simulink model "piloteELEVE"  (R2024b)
settings: Solver=ode45  StartTime=0.0  StopTime=35*45*12  RelTol=1e-3  EnableMultiTasking=on
PreLoadFcn:
  | M=0
InitFcn:
  | modelename = gcs
  | path = strcat(gcs,'/mecanisme pilote/Mass')
  | if M==0
  |     set_param(path,'Commented','on')
  | else
  |     set_param(path,'Commented','off')
  | end
libraries: fl_lib x14, nesl_utility x5, sdl_lib x1

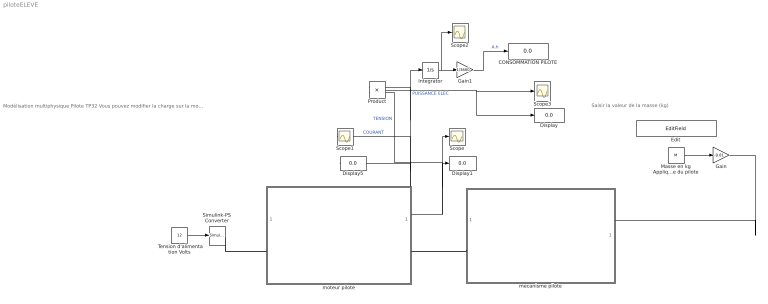
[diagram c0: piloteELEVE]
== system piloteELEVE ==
  note: Saisir la valeur de la masse (kg)
  note: Modélisation multiphysique Pilote TP32 Vous pouvez modifier la charge sur la motorisation du pilote en modifiant la valeur de la masse appliquée sur la tige du pilote.
  " Tension d'alimentation Volts" : Constant  Value=12
  CONSOMMATION PILOTE : Display
  Display : Display
  Display1 : Display
  Display5 : Display
  Edit : EditField  LabelPosition=Hide  ShowInitialText=on  Alignment=Center
  Gain : Gain  Gain=-9.81
  Gain1 : Gain  Gain=1/3600
  Integrator : Integrator
  Masse en kg Appliquée sur la tige en sortie du pilote : Constant  Value=M
  Product : Product
  Scope{,1..3} (4 alike) : Scope
  Simulink-PS Converter : nesl_utility/Simulink-PS Converter  PhysicalDomain=network_engine_domain  SubClassName=ps_input  LeftPortType=input  RightPortType=output  PseudoPeriodic=off  Frequencies=[]  NoiseDistribution=none  NoiseParameters=[]  Unit=1  AffineConversion=off  FilteringAndDerivatives=zero  SimscapeFilterOrder=1  InputFilterTimeConstant=0.001  UdotUserProvided=1
  mecanisme pilote : Subsystem
  moteur pilote : Subsystem
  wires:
  " Tension d'alimentation Volts"/1 -> Simulink-PS Converter/1
  Masse en kg Appliquée sur la tige en sortie du pilote/1 -> Gain/1
  Gain/1 -> mecanisme pilote/1(Masse accrochée sur la tige)
  Integrator/1 -> Scope2/1, Gain1/1
  Product/1 -> Display/1, Scope3/1  "PUISSANCE ELEC"
  Gain1/1 -> CONSOMMATION PILOTE/1  "A.h"
  moteur pilote/2(TENSION) -> Display1/1, Scope/1, Product/2  "TENSION"
  moteur pilote/1(COURANT) -> Display5/1, Integrator/1, Product/1, Scope1/1  "COURANT"
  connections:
  Simulink-PS Converter/RConn1 -- moteur pilote/LConn1
  moteur pilote/RConn1 -- mecanisme pilote/LConn1

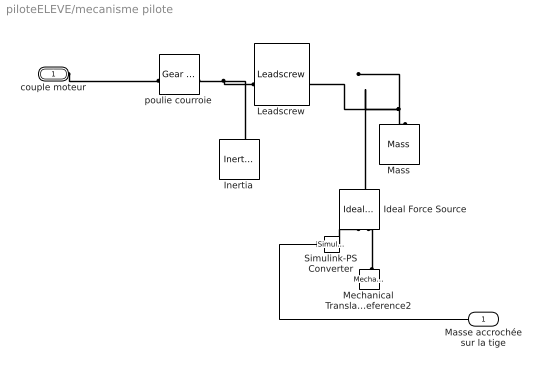
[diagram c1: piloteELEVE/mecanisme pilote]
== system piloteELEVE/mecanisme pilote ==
  Masse accrochée sur la tige : Inport
  Ideal Force Source : fl_lib/Mechanical/Mechanical Sources/Ideal Force Source
  Inertia : fl_lib/Mechanical/Rotational Elements/Inertia  inertia=0.0015 kg*m^2  num_ports=foundation.enum.numPorts2.one  w_specify=off  w_priority=High  w=0 rad/s  w_nominal_specify=off  w_nominal_value=1  w_nominal_unit=rad/s  t_specify=off  t_priority=None  t=0 N*m  t_nominal_specify=off  t_nominal_value=1  t_nominal_unit=N*m
  Leadscrew : sdl_lib/Gears/Rotational- Translational/Leadscrew  Lead=0.003 m  helix_type=sdl.enum.handedness.right  friction_model=sdl.enum.gear_friction.constant  friction_parameterization=sdl.enum.frictionParameterization.geometry  lambda=15 deg  alpha=14.5 deg  fr_coeff=0.25  eff_sn=0.75  eff_ns=0.45  temperature_TLU=[280, 300, 320] K  efficiency_sn_TLU=[.75, .65, .6]  efficiency_ns_TLU=[.5, .45, .4]  pwr_thr=0.001 W  mu_visc=0.0008 N*m*s/rad  thermal_mass=50 J/K  temperature_specify=off  temperature_priority=High  temperature=300 K  temperature_nominal_specify=off  temperature_nominal_value=1  temperature_nominal_unit=K
  Mass : fl_lib/Mechanical/Translational Elements/Mass  mass=M kg  num_ports=foundation.enum.numPorts2.one  v_specify=off  v_priority=High  v=0 m/s  v_nominal_specify=off  v_nominal_value=1  v_nominal_unit=m/s  f_specify=off  f_priority=None  f=0 N  f_nominal_specify=off  f_nominal_value=1  f_nominal_unit=N
  Mechanical Translational Reference2 : fl_lib/Mechanical/Translational Elements/Mechanical Translational Reference
  Simulink-PS Converter : nesl_utility/Simulink-PS Converter  PhysicalDomain=network_engine_domain  SubClassName=ps_input  LeftPortType=input  RightPortType=output  PseudoPeriodic=off  Frequencies=[]  NoiseDistribution=none  NoiseParameters=[]  Unit=1  AffineConversion=off  FilteringAndDerivatives=provide  SimscapeFilterOrder=1  InputFilterTimeConstant=0.001  UdotUserProvided=0
  poulie courroie : fl_lib/Mechanical/Mechanisms/Gear Box  ratio=71/20  t_in_specify=off  t_in_priority=None  t_in=0 N*m  t_in_nominal_specify=off  t_in_nominal_value=1  t_in_nominal_unit=N*m  t_out_specify=off  t_out_priority=None  t_out=0 N*m  t_out_nominal_specify=off  t_out_nominal_value=1  t_out_nominal_unit=N*m
  couple moteur : PMIOPort  Side=Left
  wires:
  Masse accrochée sur la tige/1 -> Simulink-PS Converter/1
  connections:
  Mass/LConn1 -- Leadscrew/RConn1 -- Ideal Force Source/LConn1
  couple moteur/RConn1 -- poulie courroie/LConn1
  poulie courroie/RConn1 -- Inertia/LConn1 -- Leadscrew/LConn1
  Simulink-PS Converter/RConn1 -- Ideal Force Source/RConn1
  Mechanical Translational Reference2/LConn1 -- Ideal Force Source/RConn2

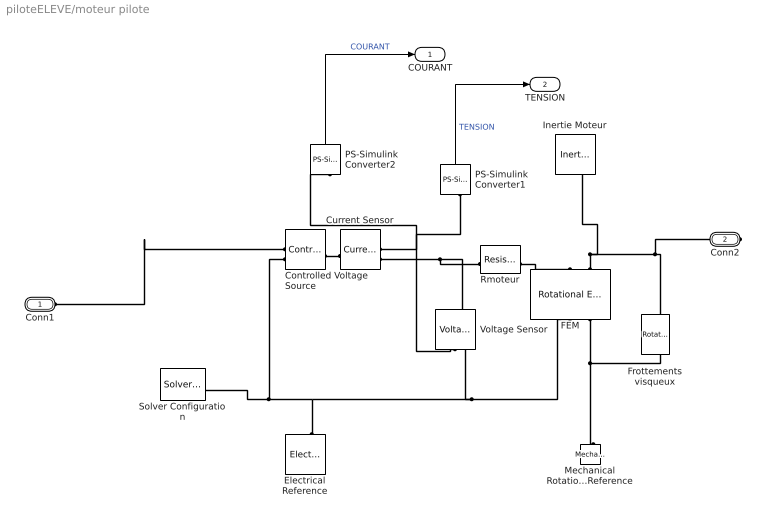
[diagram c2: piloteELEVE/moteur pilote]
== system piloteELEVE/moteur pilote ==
  Controlled Voltage Source : fl_lib/Electrical/Electrical Sources/Controlled Voltage Source
  Current Sensor : fl_lib/Electrical/Electrical Sensors/Current Sensor
  Electrical Reference : fl_lib/Electrical/Electrical Elements/Electrical Reference
  FEM : fl_lib/Electrical/Electrical Elements/Rotational Electromechanical Converter  K=1 V/(rad/s)  i_specify=off  i_priority=None  i=0 A  i_nominal_specify=off  i_nominal_value=1  i_nominal_unit=A  v_specify=off  v_priority=None  v=0 V  v_nominal_specify=off  v_nominal_value=1  v_nominal_unit=V  t_specify=off  t_priority=None  t=0 N*m  t_nominal_specify=off  t_nominal_value=1  t_nominal_unit=N*m  w_specify=off  w_priority=None  w=0 rad/s  w_nominal_specify=off  w_nominal_value=1  w_nominal_unit=rad/s
  Frottements visqueux : fl_lib/Mechanical/Rotational Elements/Rotational Damper  D=1 N*m*s/rad  w_specify=off  w_priority=None  w=0 rad/s  w_nominal_specify=off  w_nominal_value=1  w_nominal_unit=rad/s  t_specify=off  t_priority=None  t=0 N*m  t_nominal_specify=off  t_nominal_value=1  t_nominal_unit=N*m
  Inertie Moteur : fl_lib/Mechanical/Rotational Elements/Inertia  inertia=1 kg*m^2  num_ports=foundation.enum.numPorts2.one  w_specify=on  w_priority=High  w=0 rad/s  w_nominal_specify=off  w_nominal_value=1  w_nominal_unit=rad/s  t_specify=off  t_priority=None  t=0 N*m  t_nominal_specify=off  t_nominal_value=1  t_nominal_unit=N*m
  Mechanical Rotational Reference : fl_lib/Mechanical/Rotational Elements/Mechanical Rotational Reference
  PS-Simulink Converter1 : nesl_utility/PS-Simulink Converter  PhysicalDomain=network_engine_domain  SubClassName=ps_output  LeftPortType=input  RightPortType=output  PseudoPeriodic=off  Frequencies=[]  VectorFormat=1-D array  Unit=V  AffineConversion=off
  PS-Simulink Converter2 : nesl_utility/PS-Simulink Converter  PhysicalDomain=network_engine_domain  SubClassName=ps_output  LeftPortType=input  RightPortType=output  PseudoPeriodic=off  Frequencies=[]  VectorFormat=1-D array  Unit=A  AffineConversion=off
  Rmoteur : fl_lib/Electrical/Electrical Elements/Resistor  R=1 Ohm  i_specify=off  i_priority=None  i=0 A  i_nominal_specify=off  i_nominal_value=1  i_nominal_unit=A  v_specify=off  v_priority=None  v=0 V  v_nominal_specify=off  v_nominal_value=1  v_nominal_unit=V
  Solver Configuration : nesl_utility/Solver Configuration  PhysicalDomain=network_engine_domain  SubClassName=solver  LeftPortType=input  RightPortType=generic  Tones=[]  Harmonics=[]  SimulateNoise=off  Profile=off  UseLocalSampling=off  EnableSwitchedLinearOptims=on  FrequencyDomain=off  UseCCode=off  RelTol=0.001  AbsTol=1e-06  MinStep=1e-09  ToWorkspace=off  RevertToSquareIcSolve=off  NumHomotopyIterations=100  PhasorMode=off  PhasorModeNumHarmonics=1  ConsistencySolver=NEWTON_FTOL  IndexReductionMethod=DerivativeReplacement  DoDC=off  ResidualTolerance=1e-09  ConsistencyTolSource=GLOBAL  ConsistencyAbsTol=0.001  ConsistencyRelTol=0.001  ConsistencyTolFactor=0.001  UseLocalSolver=off  LocalSolverChoice=NE_BACKWARD_EULER_ADVANCER  ResolveIndetEquations=on  FunctionEvalNumThread=1  LocalSolverSampleTime=0.001  DoFixedCost=off  MaxNonlinIter=3  MaxModeIter=2  ComputeImpulses=off  ImpulseIterations=2  LinearAlgebra=Sparse  LinearAlgebraNumThread=0  EquationFormulation=NE_TIME_EF  DelaysMemoryBudget=1024  AutomaticFiltering=on  FilteringTimeConstant=0.001  PartitionStorageMethod=AS_NEEDED  PartitionMemoryBudget=1024  PartitionMethod=FAST  MultibodyUseLocalSolver=off  MultibodyLocalSolverChoice=ODE1  MultibodyLocalSolverSampleTime=0.001
  Voltage Sensor : fl_lib/Electrical/Electrical Sensors/Voltage Sensor
  Conn1 : PMIOPort  Side=Left
  Conn2 : PMIOPort  Port=2  Side=Right
  COURANT : Outport
  TENSION : Outport  Port=2
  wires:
  PS-Simulink Converter1/1 -> TENSION/1  "TENSION"
  PS-Simulink Converter2/1 -> COURANT/1  "COURANT"
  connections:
  Electrical Reference/LConn1 -- Solver Configuration/RConn1 -- Controlled Voltage Source/RConn2 -- Voltage Sensor/RConn2 -- FEM/RConn1
  Rmoteur/RConn1 -- FEM/LConn1
  PS-Simulink Converter1/LConn1 -- Voltage Sensor/RConn1
  Current Sensor/RConn1 -- PS-Simulink Converter2/LConn1
  FEM/LConn2 -- Inertie Moteur/LConn1 -- Frottements visqueux/LConn1 -- Conn2/RConn1
  FEM/RConn2 -- Frottements visqueux/RConn1 -- Mechanical Rotational Reference/LConn1
  Current Sensor/RConn2 -- Rmoteur/LConn1 -- Voltage Sensor/LConn1
  Current Sensor/LConn1 -- Controlled Voltage Source/LConn1
  Conn1/RConn1 -- Controlled Voltage Source/RConn1
